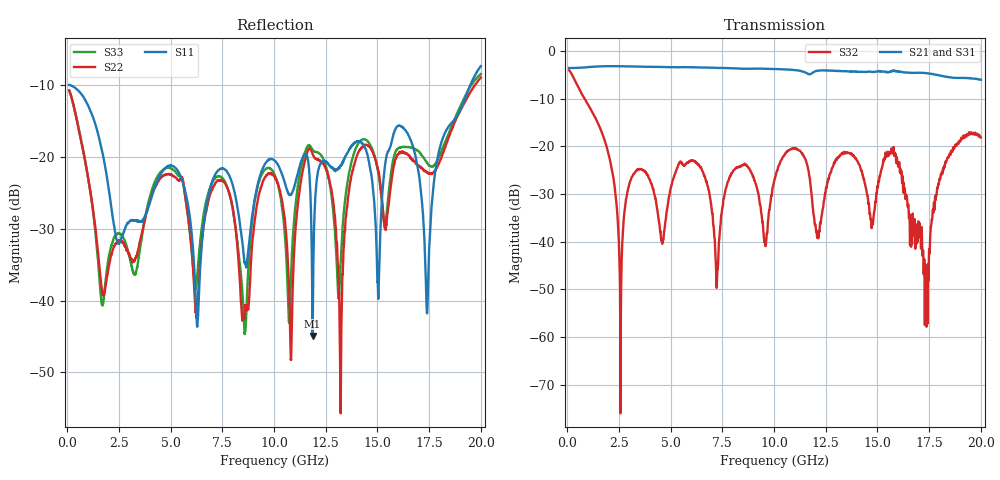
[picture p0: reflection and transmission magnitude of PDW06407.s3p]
!The following data was pulled from an Agilent PNA
!This sNp file was generated from the data in the RF Test software
!NOTE:  Smoothing/Math/Corrections applied on any given trace ARE included in the data saved here
# MHz S dB R 50
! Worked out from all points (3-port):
!   6401 points, 100 MHz to 20 GHz, reference 50 ohm
!   strongest paths, dB at 100 MHz, 5.075 GHz, 10.05 GHz, 15.03 GHz, 20 GHz:
!     S21: -3.6, -3.4, -3.8, -4.3, -6.1
!     S31: -3.6, -3.4, -3.8, -4.4, -6.5
!     S32: -4.1, -27.6, -26.6, -28.5, -18.2
!   lowest |S11| = -44.9 dB at 11.87 GHz (marker M1), VSWR 1.01, Z = 50.6 + j0.125 ohm
!   |S11| at or under -10 dB: 181.4 MHz to 19.48 GHz (19.3 GHz wide, 196 % of centre)
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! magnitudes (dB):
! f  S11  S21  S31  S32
! 100 MHz  -9.9  -3.6  -3.6  -4.1
! 2.587 GHz  -31.6  -3.2  -3.2  -69.0
! 3.415 GHz  -29.0  -3.3  -3.3  -24.9
! 10.05 GHz  -20.5  -3.8  -3.8  -26.6
! 10.82 GHz  -25.3  -4.0  -4.0  -20.6
! 11.87 GHz  -44.9  -4.6  -4.6  -32.3
! 13.21 GHz  -21.2  -4.2  -4.4  -21.9
! 15.75 GHz  -17.2  -4.3  -4.0  -21.5
! 17.38 GHz  -41.0  -4.7  -4.7  -57.8
! 20 GHz  -7.3  -6.1  -6.5  -18.2
